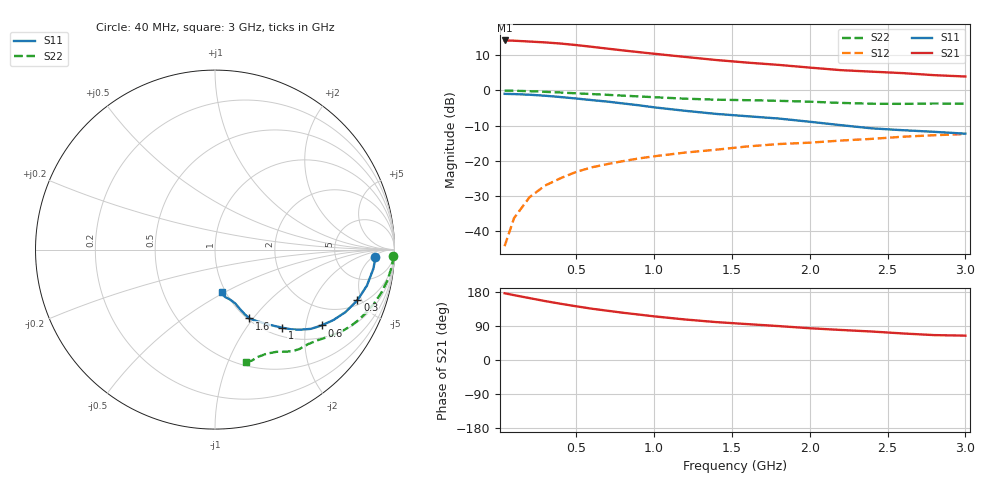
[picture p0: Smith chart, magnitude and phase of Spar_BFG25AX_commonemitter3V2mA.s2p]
! Filename:  BFG25AXJ.S2P  Version:  2.0
! NXP part #: BFG25A/X  Date: May 1990
! Bias condition: Vce=3.0V, Ic=2.0mA
#  MHz  S  MA  R  50
! Freq  S11  S21  S12  S22  !GUM [dB]
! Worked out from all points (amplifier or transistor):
!   21 points, 40 MHz to 3 GHz, reference 50 ohm
!   highest |S21| = 14.3 dB at 40 MHz (marker M1)
!   |S21| within 3 dB of that: start of sweep to 833.2 MHz
!   unconditionally stable (mu >= 1): nowhere
!   at 300 MHz: K = 0.20, MSG = 20.4 dB, |S12| = -27.1 dB
!   at 1 GHz: K = 0.55, MSG = 14.6 dB, |S12| = -18.8 dB
!   at 3 GHz: K = 0.92, MSG = 8.2 dB, |S12| = -12.4 dB
!   lowest NFmin = 2.30 dB at 500 MHz
!   S11 on the Smith chart (normalised r, x): 40 MHz: 15, -6; 300 MHz: 2.38, -4.61; 600 MHz: 1.37, -2.46; 1 GHz: 1.16, -1.50; 1.6 GHz: 1.02, -0.96; 3 GHz: 0.96, -0.49
40  0.895 -2.6  5.176 176.1  0.006 88.6  0.995 -2.0
100  0.889 -6.8  5.134 171.2  0.015 85.4  0.991 -5.0
200  0.87 -13.3  4.996 163.3  0.03 81.3  0.977 -9.9
300  0.842 -19.6  4.854 155.5  0.044 77.6  0.957 -14.6
400  0.806 -25.6  4.677 148.4  0.056 74.4  0.935 -18.9
500  0.768 -30.7  4.447 141.7  0.069 71.6  0.911 -22.8
600  0.729 -35.4  4.202 135.4  0.08 69.6  0.889 -26.4
700  0.694 -39.5  3.958 130.0  0.089 67.3  0.867 -29.5
800  0.653 -43.1  3.733 124.7  0.098 66.2  0.845 -32.2
900  0.616 -46.2  3.53 120.0  0.107 64.4  0.823 -34.6
1000  0.575 -49.2  3.344 115.2  0.115 62.7  0.802 -37.0
1200  0.513 -54.5  3.012 106.9  0.13 59.7  0.764 -41.3
1400  0.463 -59.5  2.722 100.0  0.143 58.6  0.739 -45.5
1600  0.429 -63.4  2.498 94.7  0.159 57.0  0.727 -49.6
1800  0.398 -65.2  2.319 89.5  0.172 55.4  0.712 -52.6
2000  0.358 -67.3  2.122 83.8  0.18 53.7  0.692 -55.3
2200  0.32 -69.4  1.951 79.3  0.193 52.2  0.665 -58.9
2400  0.288 -73.7  1.856 75.1  0.204 50.2  0.647 -63.7
2600  0.271 -77.7  1.769 70.0  0.219 47.9  0.644 -68.5
2800  0.257 -80.0  1.654 65.7  0.23 46.8  0.652 -71.8
3000  0.242 -80.5  1.583 64.3  0.239 46.2  0.649 -74.4
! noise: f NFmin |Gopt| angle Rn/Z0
500  2.3  0.79  5  2.3
1000  2.3  0.74  14  2.5
2000  2.8  0.7  37  1.8
